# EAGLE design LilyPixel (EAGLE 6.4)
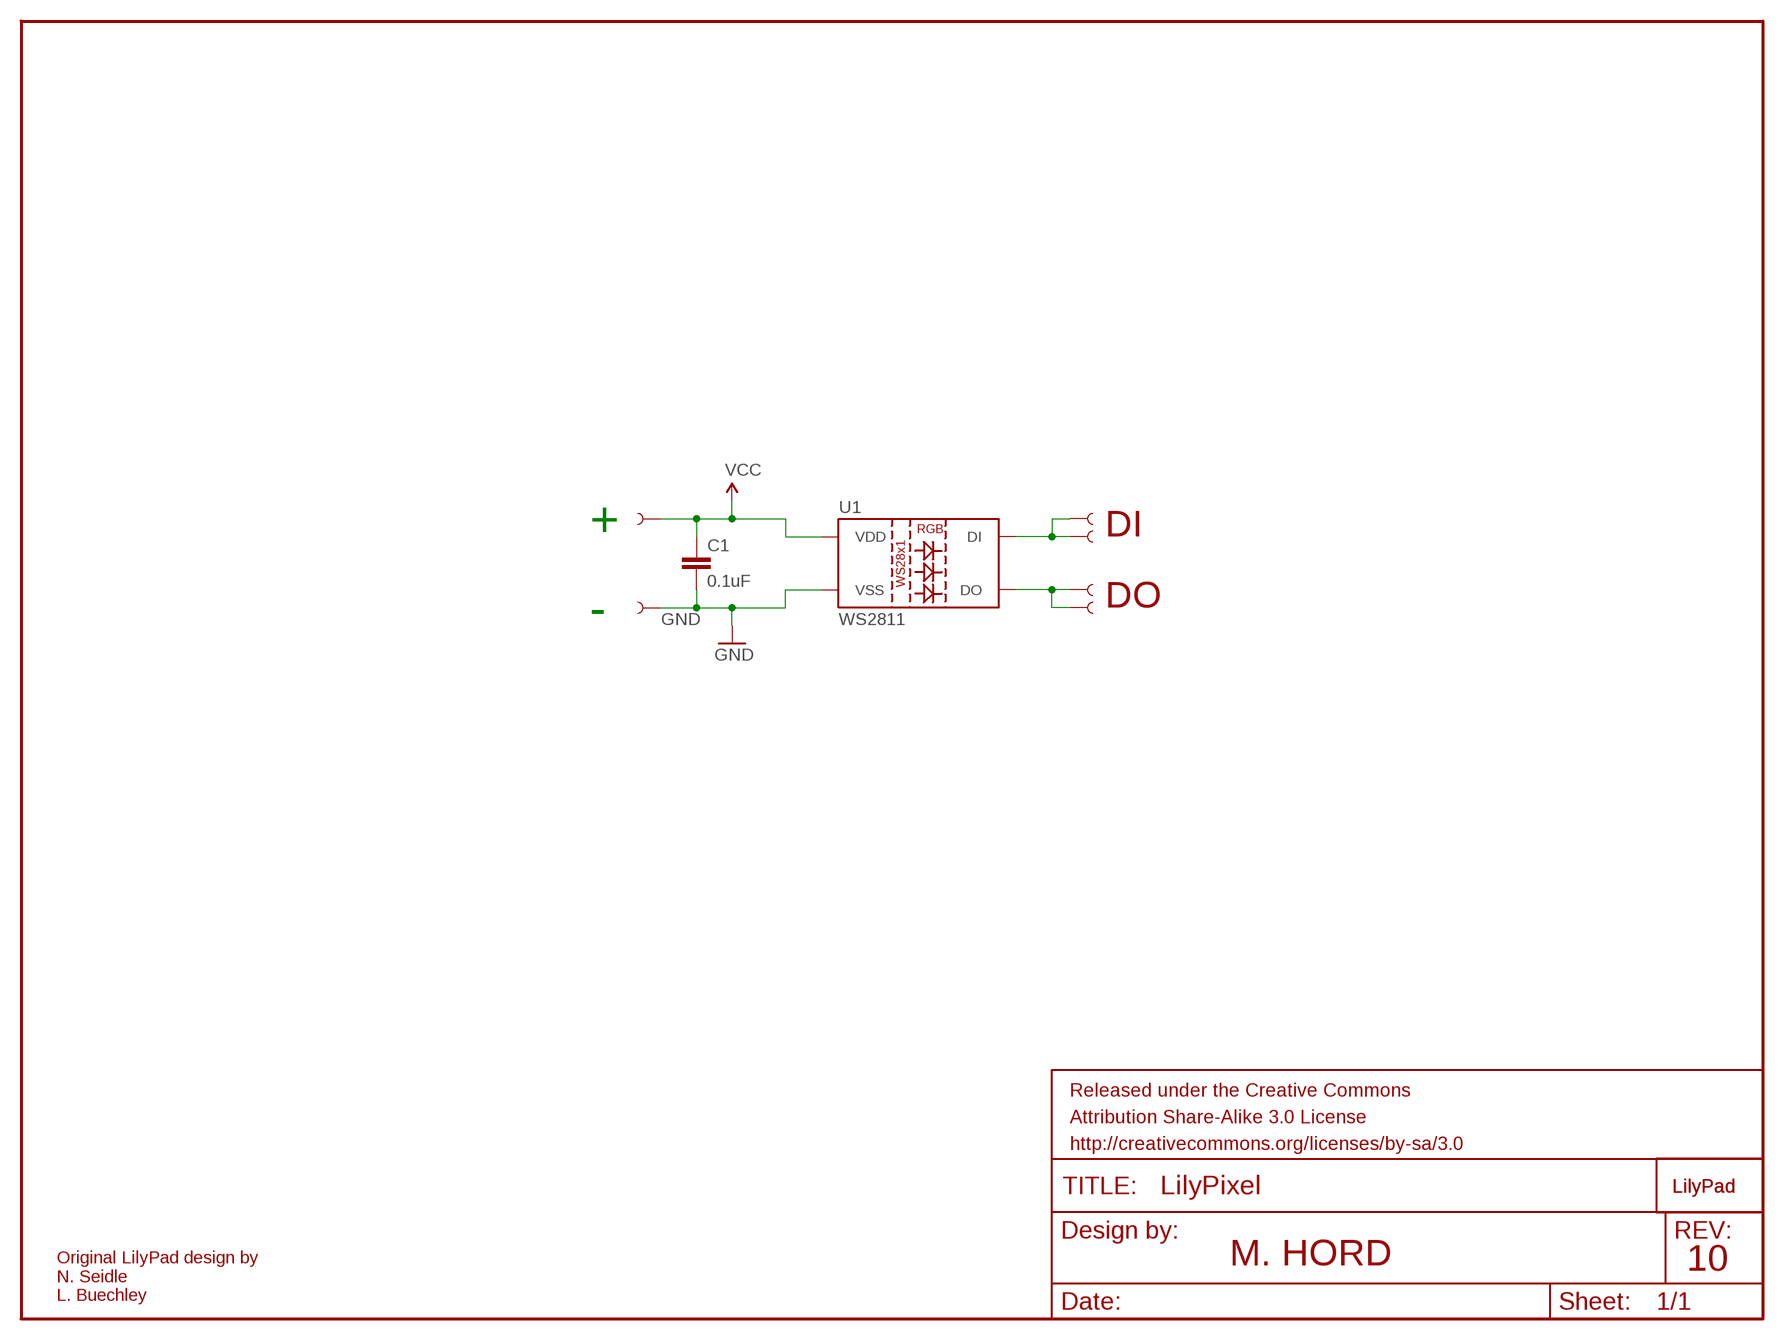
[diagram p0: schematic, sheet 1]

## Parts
C1  0.1uF  0.1UF-25V(+80/-20%)(0603)  [0603-CAP]
FRAME1  FRAME-LETTER  [CREATIVE_COMMONS]
U1  WS2811  LED-TRICOLOR-5050-ICWS2811  [LED-TRICOLOR-5050-IC]
U$1  LOGO-LPLP  [LOGO-LILYPAD]
U$2  SEWTAP6  [PETAL-SMALL-2SIDE]
U$3  SEWTAP6  [PETAL-SMALL-2SIDE]
U$4  SEWTAP6  [PETAL-SMALL-2SIDE]
U$5  SEWTAP6  [PETAL-SMALL-2SIDE]
U$6  SEWTAP6  [PETAL-SMALL-2SIDE]
U$7  SEWTAP6  [PETAL-SMALL-2SIDE]
U$8  LOGO-LPL  [LOGO-L]

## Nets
DI: U1.2(DI) U$2.1 U$4.1
DO: U1.1(DO) U$3.1 U$5.1
GND: C1.2 U1.6(VSS) U$7.1
VCC: C1.1 U1.3(VDD) U1.5(VDD) U$6.1

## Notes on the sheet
- + | DI
- DO
- -
- M. HORD | 10
- Original LilyPad design by
  N. Seidle
  L. Buechley

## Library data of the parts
C1 = SparkFun-Capacitors:0.1UF-25V(+80/-20%)(0603): Ceramic; PROD_ID: CAP-00810
FRAME1 = SparkFun-Aesthetics:FRAME-LETTER: Schematic Frame
U1 = SparkFun-LED:LED-TRICOLOR-5050-IC: WS2811 RGB LED w/driver 5x5mm SMD LED with built-in controller IC. DIO-11598; PROD_ID: DIO-11598
U$1 U$8 = LilyPad-Wearables:LOGO-LP
U$2-U$7 = LilyPad-Wearables:SEWTAP

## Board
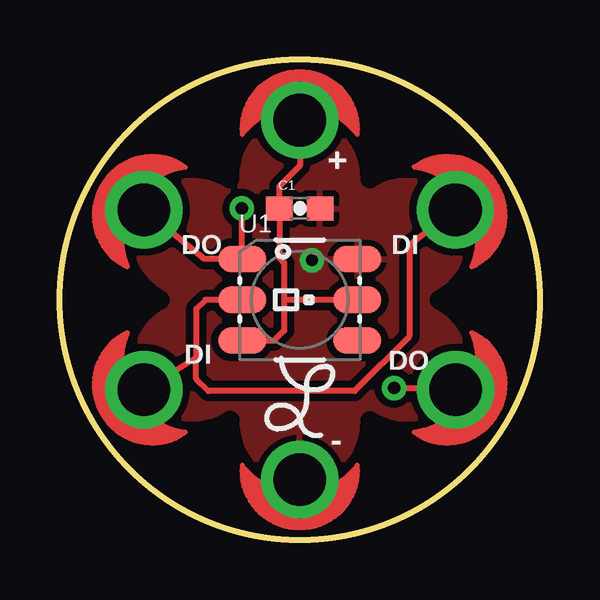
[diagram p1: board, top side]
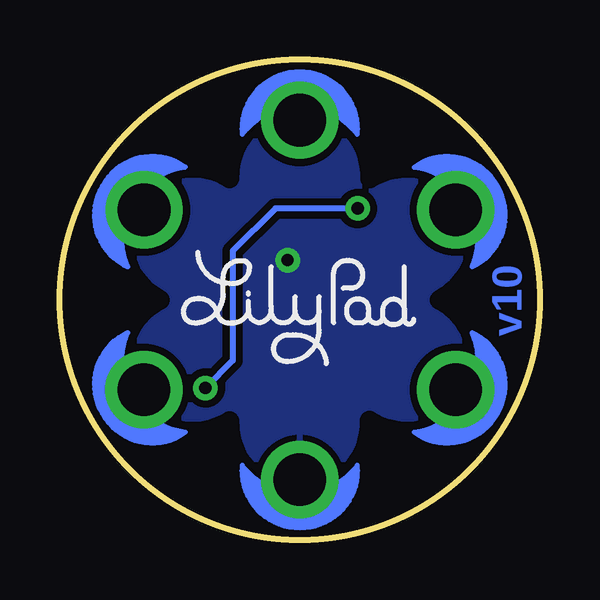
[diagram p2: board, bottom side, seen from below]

Size 20 x 20 mm. Coordinates in mm from the lower left corner, seen from the top.
Outline: circle at 10,10 radius 10
Copper layers (1*16): Top 0.035mm / dielectric 1.5mm / Bottom 0.035mm
Design rules "Sparkfun": minimum track width 8mil, minimum drill 20mil, track to track 8mil, track to pad 8mil, pad to pad 8mil, via to via 8mil, smd to smd 8mil, copper to edge 8mil, drill to drill 8mil, minimum pad ring 12mil, minimum via ring 10mil, stop-mask expansion 4mil, vias tented up to drill 20mil, thermal gap 10mil
tRestrict: area -0.1,10 to 10,20; area 10,10 to 20.1,20; area 10,-0.1 to 20.1,10; area -0.1,-0.1 to 10,10; 6 lines
bRestrict: area -0.1,10 to 10,20; area 10,10 to 20.1,20; area 10,-0.1 to 20.1,10; area -0.1,-0.1 to 10,10; 6 lines

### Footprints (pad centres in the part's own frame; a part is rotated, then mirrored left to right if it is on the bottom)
0603-CAP = smd 1.1 x 1: 1 -0.85,0; 2 0.85,0
LED-TRICOLOR-5050-IC = smd 2 x 1.1: 1 -2.4,1.7; 2 -2.4,0; 3 -2.4,-1.7; 4 2.4,-1.7; 5 2.4,0; 6 2.4,1.7
PETAL-SMALL-2SIDE = drill 2.2: 1 0,0

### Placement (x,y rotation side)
C1  10,13.81 0 top
FRAME1  not placed on the board
U1  10,10 0 top
U$1  10,10 0 bottom
U$2  3.5,6.25 300 top
U$3  16.5,6.25 60 top
U$4  16.49,13.75 120 top
U$5  3.5,13.75 240 top
U$6  10,17.49 180 top
U$7  10,2.5 0 top
U$8  10,5.94 0 top

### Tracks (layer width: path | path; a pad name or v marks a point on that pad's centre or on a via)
DI
  Top 0.254: U$2.1 5.68,7.59 | U1.2 6.06,10 5.68,9.62 5.68,7.59 | U$4.1 14.57,12.29 14.57,8.48 12.29,6.19 6.19,6.19 5.68,6.7 5.68,7.59
DO  (via drill 0.51)
  Top 0.254: U$5.1 5.94,11.78 6.01,11.7 U1.1 7.6,13.8 v7.59,13.81 | v13.94,6.32 16.43,6.32 U$3.1
  Bottom 0.254: v7.59,13.81 11.02,13.81 12.79,12.03 12.79,7.46 v13.94,6.32
GND  (via drill 0.51)
  other vias: 10.51,11.65
  pour Bottom (isolate 0.305): 1.11,18.89 1.11,1.11 18.89,1.11 18.89,18.89
  pour Top (isolate 0.305): 1.11,18.89 1.11,1.11 18.89,1.11 18.89,18.89
VCC
  Top 0.254: U$6.1 10,15.59 9.15,14.74 C1.1 9.15,11.74 9.35,11.54 9.35,10 | 9.35,10 9.35,8.71 8.94,8.3 U1.3 | U1.5 9.35,10

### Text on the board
Bottom: v10
tPlace: + | DO | DI | DI | DO | -
tValues: M. HORD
